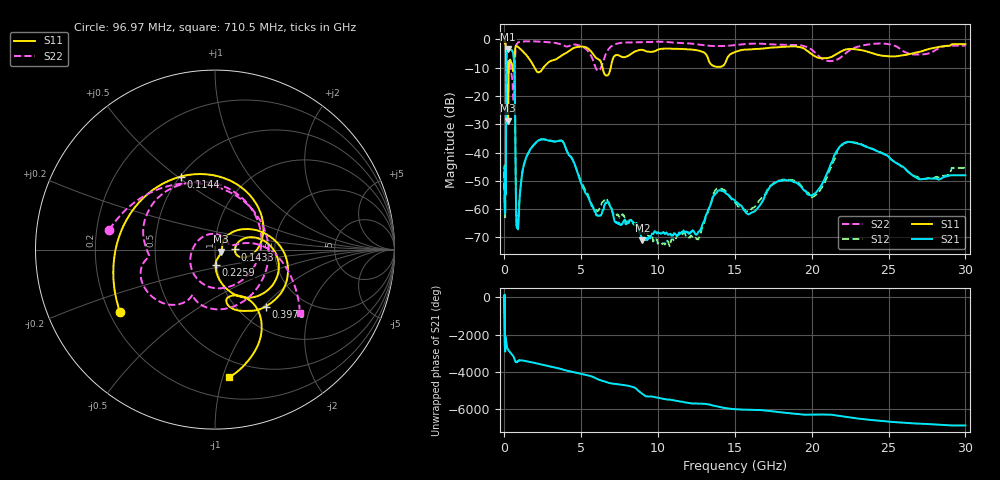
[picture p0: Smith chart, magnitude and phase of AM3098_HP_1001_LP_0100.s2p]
! Date/Time: Thu, Feb 28, 2019 8:40 AM
! Network Analyzer: Agilent Technologies E8364B Rev: A.07.50.67
! Sweep from 0.010 to 30.000 GHz, 1601 Points, Sweep Type: LOG
! Power Supply: 5.022 V, 0.002 A
# Hz S DB R 50
!freq MagS11 AngS11 MagS21 AngS21 MagS12 AngS12 MagS22 AngS22
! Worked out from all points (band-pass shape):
!   1601 points, 10 MHz to 30 GHz, reference 50 ohm
!   highest |S21| = -3.34 dB at 237.5 MHz (marker M1); lowest = -71.1 dB at 8.982 GHz (marker M2)
!   |S21| within 3 dB of the highest: 129.3 MHz to 605.6 MHz (476.3 MHz wide, 130 % of centre)
!   lowest |S11| = -28.7 dB at 237.5 MHz (marker M3), VSWR 1.08, Z = 53.6 - j1.24 ohm
!   |S11| at or under -10 dB: 199.1 MHz to 289 MHz (89.95 MHz wide, 36.9 % of centre); 1.959 GHz to 2.531 GHz (571.4 MHz wide, 25.4 % of centre); 6.382 GHz to 6.917 GHz (535.4 MHz wide, 8.05 % of centre)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
!   |S22| runs from -21.8 to -0.5 dB; largest |S21 - S12| = 0.0096
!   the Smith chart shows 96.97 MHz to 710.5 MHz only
!   S11 on the Smith chart (normalised r, x): 96.97 MHz: 0.24, -0.28; 114.4 MHz: 0.50, +0.51; 143.3 MHz: 1.25, +0.00; 225.9 MHz: 0.99, -0.17; 397.6 MHz: 1.33, -1.03; 710.5 MHz: 0.36, -1.05
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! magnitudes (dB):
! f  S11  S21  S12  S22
! 10 MHz  -0.3  -45.5  -46.2  -0.5
! 38.04 MHz  -0.5  -60.4  -59.2  -0.8
! 96.97 MHz  -4.0  -43.2  -41.9  -4.4
! 114.4 MHz  -6.9  -16.6  -16.7  -10.5
! 143.3 MHz  -19.1  -4.5  -4.5  -10.7
! 144.7 MHz  -18.9  -4.5  -4.4  -10.5
! 185.8 MHz  -8.6  -3.9  -3.9  -7.0
! 225.9 MHz  -21.4  -3.4  -3.4  -8.6
! 237.5 MHz  -28.7  -3.3  -3.3  -8.7
! 397.6 MHz  -7.4  -3.6  -3.6  -9.6
! 550.5 MHz  -11.0  -4.6  -4.6  -18.6
! 649.3 MHz  -6.4  -10.9  -10.9  -14.7
! 710.5 MHz  -2.9  -36.1  -35.9  -4.6
! 773.6 MHz  -2.3  -64.4  -62.5  -1.9
! 863.6 MHz  -2.6  -66.0  -64.5  -1.1
! 2.084 GHz  -11.2  -36.3  -36.3  -0.7
! 3.76 GHz  -5.6  -35.9  -35.9  -1.9
! 7.926 GHz  -6.1  -64.9  -63.6  -1.1
! 8.982 GHz  -3.7  -71.1  -68.2  -1.0
! 12.31 GHz  -3.7  -67.8  -70.3  -1.5
! 22.56 GHz  -3.4  -36.3  -36.3  -3.5
! 30 GHz  -1.7  -48.0  -45.4  -2.2
